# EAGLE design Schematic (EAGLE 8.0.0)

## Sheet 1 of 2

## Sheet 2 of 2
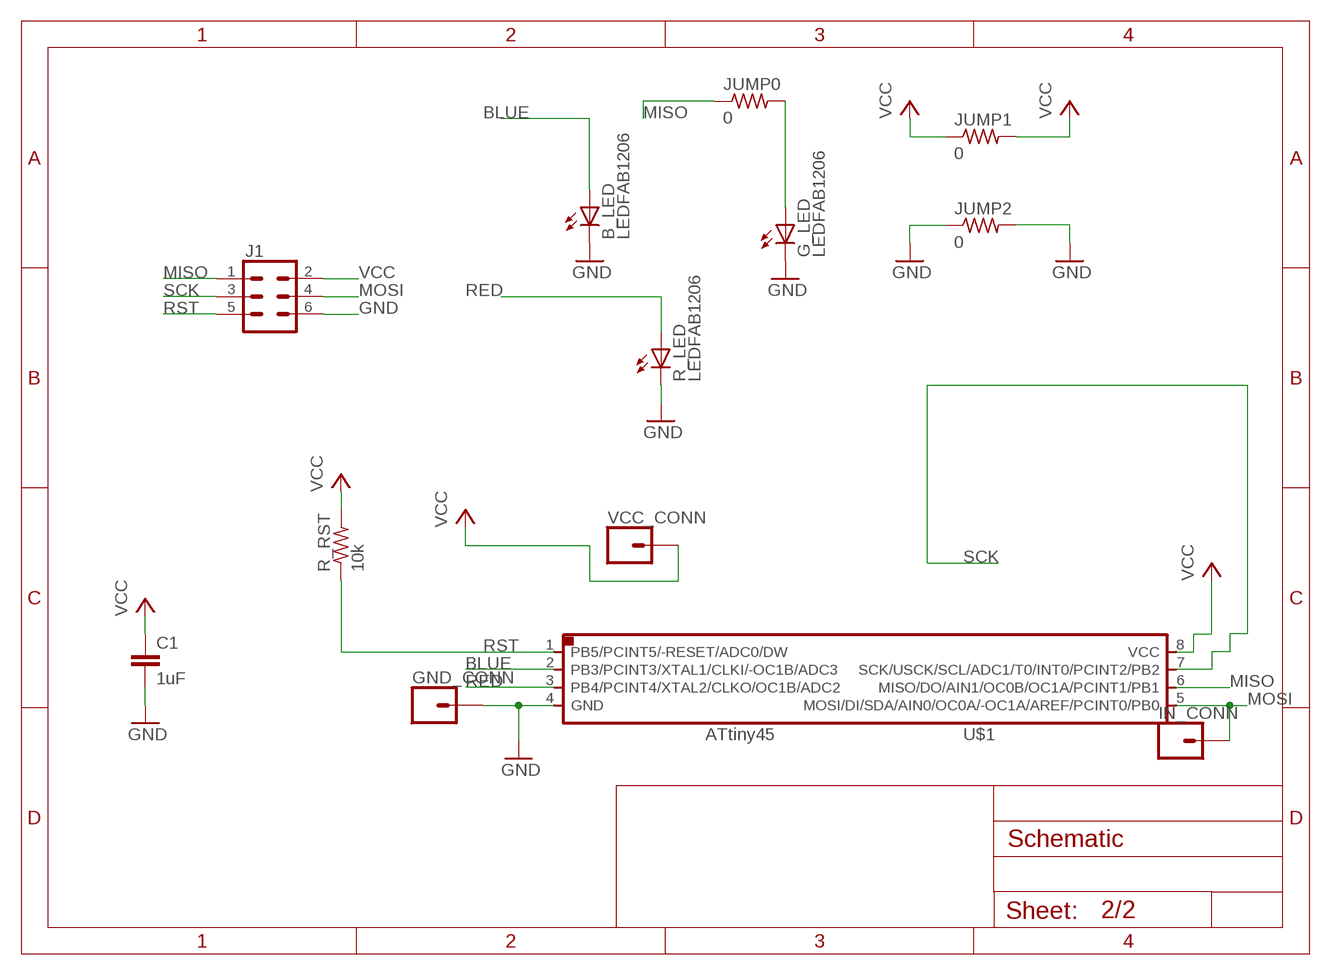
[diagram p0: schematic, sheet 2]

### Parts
B_LED  LEDFAB1206  [LED1206FAB]
C1  1uF  C-EUC1206  [C1206]
G_LED  LEDFAB1206  [LED1206FAB]
GND_CONN  CONN_01  [1X01]
IN_CONN  CONN_01  [1X01]
J1  CONN_03X2SMT  [2X3_SMT_POSTS]
JUMP0  0  RES-US1206FAB  [R1206FAB]
JUMP1  0  RES-US1206FAB  [R1206FAB]
JUMP2  0  RES-US1206FAB  [R1206FAB]
R_LED  LEDFAB1206  [LED1206FAB]
R_RST  10k  RES-US1206FAB  [R1206FAB]
U$1  ATTINY45SI  [SOIC8]
VCC_CONN  CONN_01  [1X01]

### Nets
BLUE: B_LED.1(A) U$1.2(PB3/PCINT3/XTAL1/CLKI/-OC1B/ADC3)
GND: B_LED.2(C) C1.2 G_LED.2(C) GND_CONN.1 J1.6 JUMP2.1 JUMP2.2 R_LED.2(C) U$1.4(GND)
MISO: J1.1 JUMP0.1 U$1.6(MISO/DO/AIN1/OC0B/OC1A/PCINT1/PB1)
MOSI: IN_CONN.1 J1.4 U$1.5(MOSI/DI/SDA/AIN0/OC0A/-OC1A/AREF/PCINT0/PB0)
N$1: G_LED.1(A) JUMP0.2
RED: R_LED.1(A) U$1.3(PB4/PCINT4/XTAL2/CLKO/OC1B/ADC2)
RST: J1.5 R_RST.1 U$1.1(PB5/PCINT5/-RESET/ADC0/DW)
SCK: J1.3 U$1.7(SCK/USCK/SCL/ADC1/T0/INT0/PCINT2/PB2)
VCC: C1.1 J1.2 JUMP1.1 JUMP1.2 R_RST.2 U$1.8(VCC) VCC_CONN.1

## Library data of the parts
B_LED G_LED R_LED = fab:LED: LED
C1 = rcl:C-EU: CAPACITOR, European symbol
GND_CONN IN_CONN VCC_CONN = 03_SparkFun-Connectors:CONN_01: Single connection point. Often used as Generic Header-pin footprint for 0.1 inch spaced/style header connections
J1 = SparkFun-Connectors:CONN_03X2: Multi connection point. Often used as Generic Header-pin footprint for 0.1 inch spaced/style header connections You can populate with any combo of single row headers, but if you'd like an exact match, check these: Header - 2x3 (Male, 0.1") (PRT-12807) Header - 2x3 (Female, 0.1") (PRT-13010) 2x3 Pin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; PROD_ID: CONN-11415
JUMP0 JUMP1 JUMP2 R_RST = 00_fab:RES-US: Resistor (US Symbol)
U$1 = fab:ATTINY45

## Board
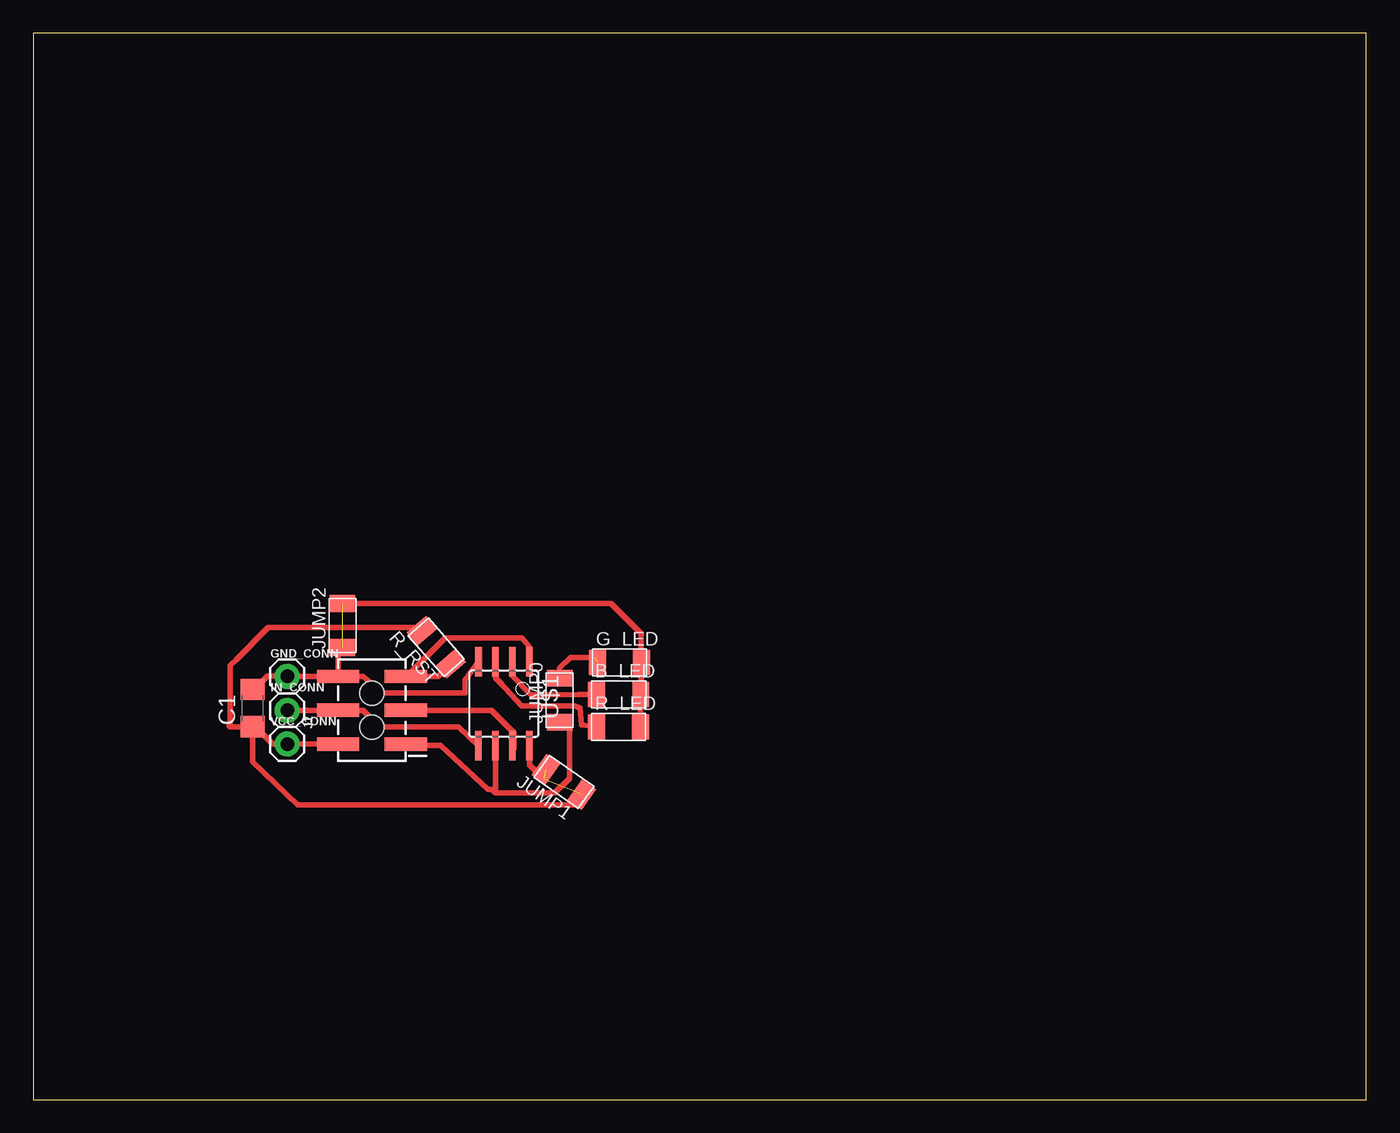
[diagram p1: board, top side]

Size 100 x 80 mm. Coordinates in mm from the lower left corner, seen from the top.
Outline: 0,0 100,0 100,80 0,80 0,0
Copper layers (1*16): Top 0.035mm / dielectric 1.5mm / Bottom 0.035mm
Design rules "default *": minimum track width 10mil, minimum drill 24mil, track to track 16mil, track to pad 16mil, pad to pad 16mil, via to via 16mil, smd to smd 16mil, copper to edge 40mil, drill to drill 16mil, minimum pad ring 10mil, minimum via ring 8mil, stop-mask expansion 4mil, vias tented up to drill 0mil, thermal gap 10mil

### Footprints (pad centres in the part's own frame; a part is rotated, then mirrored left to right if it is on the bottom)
LED1206FAB = smd 1.27 x 1.905: 1 -1.651,0; 2 1.651,0
C1206 = smd 1.6 x 1.8: 1 -1.4,0; 2 1.4,0
1X01 = drill 1.016 pad 1.88: 1 0,0
2X3_SMT_POSTS = smd 1 x 3.17: 1 -2.54,-2.54; 2 -2.54,2.54; 3 0,-2.54; 4 0,2.54; 5 2.54,-2.54; 6 2.54,2.54 | hole 1.8: -1.27,0; 1.27,0
R1206FAB = smd 1.27 x 1.905: 1 -1.651,0; 2 1.651,0
SOIC8 = smd 0.5 x 2.2: 1 -1.905,-3.154; 2 -0.645,-3.154; 3 0.625,-3.154; 4 1.895,-3.154; 5 1.905,3.154; 6 0.635,3.154; 7 -0.635,3.154; 8 -1.905,3.154

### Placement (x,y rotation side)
B_LED  43.92,30.39 0 top
C1  16.45,29.37 90 top
G_LED  43.98,32.79 0 top
GND_CONN  19.05,31.75 0 top
IN_CONN  19.05,29.21 0 top
J1  25.4,29.21 90 top
JUMP0  39.49,29.96 90 top
JUMP1  39.81,23.83 144.7 top
JUMP2  23.2,35.56 90 top
R_LED  43.91,27.95 0 top
R_RST  30.23,33.93 131 top
U$1  35.3,29.7 180 top
VCC_CONN  19.05,26.67 0 top

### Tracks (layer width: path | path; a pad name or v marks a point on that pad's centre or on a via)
BLUE
  Top 0.4: 38.39,30.37 40.93,30.38 41.81,30.38 B_LED.1 | 38.39,30.37 37.58,30.37 37.36,30.37 | 37.36,30.37 35.9,31.82 35.9,32.81 U$1.2 | 37.36,30.37 38.38,30.37 38.39,30.37
GND  (1 unrouted)
  Top 0.4: G_LED.2 45.6,30.41 B_LED.2 | 45.57,29.98 B_LED.2 | 45.57,29.98 45.57,27.18 45.56,27.16 | JUMP2.1 22.86,33.57 J1.6 GND_CONN.1 | JUMP2.2 43.34,37.21 45.63,34.92 45.6,34.88 G_LED.2 | G_LED.2 45.6,30.01 45.57,29.98 | B_LED.2 45.57,27.75 R_LED.2 | 32.4,30.51 32.4,31.45 32.39,31.46
  Top 0.406: C1.2 16.37,30.59 17.58,31.79 19.01,31.79 GND_CONN.1 | J1.6 24.76,31.75 26.28,30.51 32.4,30.51 | 32.39,31.46 U$1.4
MISO
  Top 0.4: JUMP0.1 39.41,28.23 | 39.38,28.2 JUMP0.1 | 34.59,26.47 U$1.6 34.66,23.01 34.67,23 | 40.09,28.1 JUMP0.1 | J1.1 28.05,26.57 30.56,26.57 34.12,23.26 34.42,23.26 34.67,23 | 40.08,28.09 40.09,28.1 | 34.67,23 39.12,23 39.64,23.52 39.66,23.52 40.03,23.9 40.03,23.92 40.21,24.11 40.21,27.98 40.09,28.1
MOSI
  Top 0.4: IN_CONN.1 J1.4
  Top 0.406: J1.4 24.74,29.21 25.99,27.96 31.91,27.96 U$1.5
N$1  (1 unrouted)
  Top 0.4: JUMP0.2 39.49,32.37 40.3,33.18 42.1,33.18
RED
  Top 0.4: U$1.3 34.67,31.65 35.18,31.14 35.03,31.31 36.64,29.53 40.64,29.54 41.03,29.38 41.12,28.11 R_LED.1
RST
  Top 0.406: U$1.1 37.19,32.68 37.19,33.99 36.68,34.65 30.91,34.65 28.01,31.75 J1.5 30.39,31.75 R_RST.1
SCK
  Top 0.406: J1.3 34.38,29.21 36.07,27.52 36.07,26.34 U$1.7
VCC  (2 unrouted)
  Top 0.4: R_RST.2 29.27,35.17 | C1.1 16.45,25.33 19.83,22.09 40.72,22.09 JUMP1.1 | U$1.8 37.21,26.53 37.21,25.08 37.26,25.08 38.32,24.03 | VCC_CONN.1 J1.2
  Top 0.406: VCC_CONN.1 19.04,26.68 17.94,26.68 16.84,27.79 C1.1 14.76,27.97 | 14.76,27.97 14.71,28.02 | 14.76,27.97 14.76,32.55 15.21,33 17.62,35.41 28.91,35.41 R_RST.2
